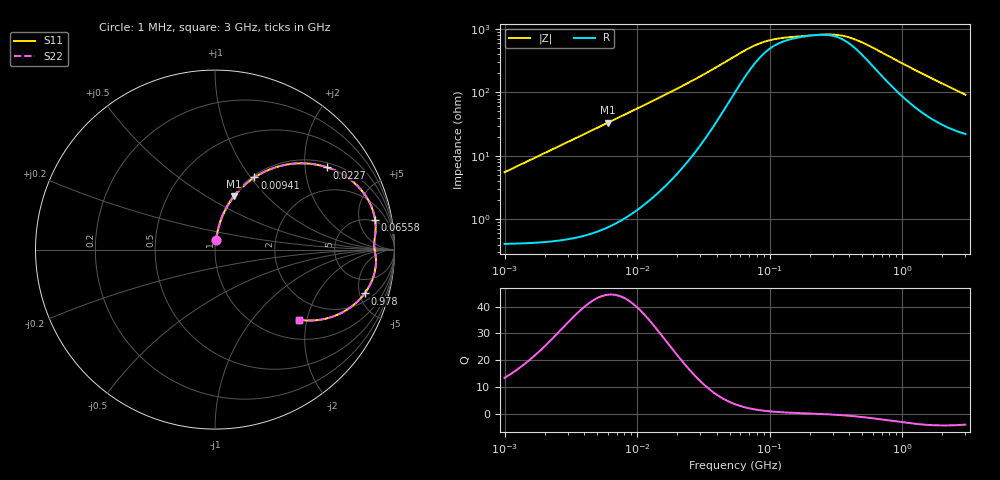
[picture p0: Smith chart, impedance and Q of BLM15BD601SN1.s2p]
! BLM15BD601SN1
# Hz S RI R 50
!Freq.(Hz) S11(Real) S11(Imag) S21(Real) S21(Imag) S12(Real) S12(Imag) S22(Real) S22(Imag)
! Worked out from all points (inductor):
!   401 points, 1 MHz to 3 GHz, reference 50 ohm
!   read as one part in series: L = 876 nH near 1.041 MHz
!   highest Q = 44.5 at 6.058 MHz (marker M1), where L = 879 nH
!   self-resonance near 226.7 MHz
!   S11 on the Smith chart (normalised r, x): 1 MHz: 1.01, +0.11; 9.41 MHz: 1.03, +1.04; 22.7 MHz: 1.14, +2.62; 65.58 MHz: 4.59, +8.52; 978 MHz: 2.81, -5.60; 3 GHz: 1.44, -1.79
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1000000  0.00706 0.0544  0.9929 -0.0544  0.9929 -0.0544  0.00706 0.0544
2055611  0.0169 0.1108  0.9831 -0.1108  0.9831 -0.1108  0.0169 0.1108
3823119  0.0472 0.1997  0.9528 -0.1997  0.9528 -0.1997  0.0472 0.1997
6058321  0.1061 0.2969  0.8939 -0.2969  0.8939 -0.2969  0.1061 0.2969
9410094  0.22 0.4022  0.78 -0.4022  0.78 -0.4022  0.22 0.4022
1.461624e7  0.4055 0.4749  0.5945 -0.4749  0.5945 -0.4749  0.4055 0.4749
1.821614e7  0.516 0.4798  0.484 -0.4798  0.484 -0.4798  0.516 0.4798
2.270269e7  0.6255 0.458  0.3745 -0.458  0.3745 -0.458  0.6255 0.458
3.526298e7  0.7991 0.3494  0.2009 -0.3494  0.2009 -0.3494  0.7991 0.3494
5.477226e7  0.8814 0.2125  0.1186 -0.2125  0.1186 -0.2125  0.8814 0.2125
6.558369e7  0.8923 0.164  0.1077 -0.164  0.1077 -0.164  0.8923 0.164
8.338914e7  0.8949 0.112  0.1051 -0.112  0.1051 -0.112  0.8949 0.112
1.039275e8  0.8919 0.0767  0.1081 -0.0767  0.1081 -0.0767  0.8919 0.0767
2.094008e8  0.8882 0.00711  0.1118 -0.00711  0.1118 -0.00711  0.8882 0.00711
2.942768e8  0.8935 -0.0263  0.1065 0.0263  0.1065 0.0263  0.8935 -0.0263
3.817355e8  0.8965 -0.0593  0.1035 0.0593  0.1035 0.0593  0.8965 -0.0593
4.951867e8  0.8944 -0.1007  0.1056 0.1007  0.1056 0.1007  0.8944 -0.1007
8.005644e8  0.8628 -0.1981  0.1372 0.1981  0.1372 0.1981  0.8628 -0.1981
9.779672e8  0.8338 -0.2441  0.1662 0.2441  0.1662 0.2441  0.8338 -0.2441
1.347129e9  0.7618 -0.3166  0.2382 0.3166  0.2382 0.3166  0.7618 -0.3166
1.855641e9  0.6572 -0.3729  0.3428 0.3729  0.3428 0.3729  0.6572 -0.3729
3e9  0.4664 -0.3904  0.5336 0.3904  0.5336 0.3904  0.4664 -0.3904
